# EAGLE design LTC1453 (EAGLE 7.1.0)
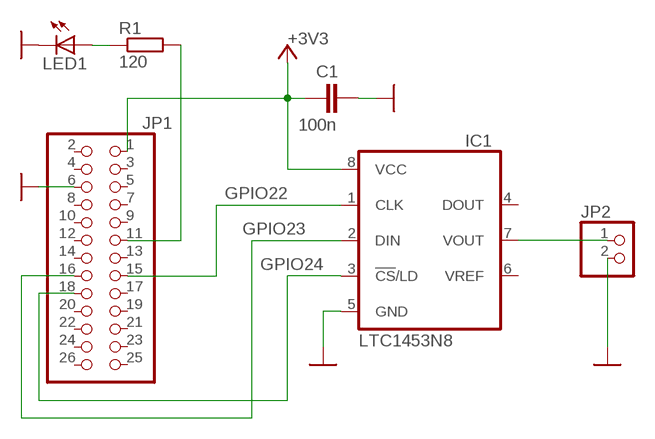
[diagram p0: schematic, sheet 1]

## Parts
C1  100n  C-EU025-024X044  [C025-024X044]
IC1  LTC1453N8  [DIL08]
JP1  PINHD-2X13  [2X13]
JP2  PINHD-1X2  [1X02]
LED1  LED5MM  [LED5MM]
R1  120  R-EU_0207/10  [0207/10]

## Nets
+3V3: C1.1 IC1.8(VCC) JP1.1
GND: C1.2 IC1.5(GND) JP1.6 JP2.2 LED1.K(C)
N$1: IC1.7(VOUT) JP2.1
N$3: IC1.3(!CS!/LD) JP1.18
N$4: IC1.1(CLK) JP1.15
N$5: IC1.2(DIN) JP1.16
N$6: LED1.A R1.1
N$7: JP1.11 R1.2
Unconnected: IC1.4(DOUT) IC1.6(VREF) JP1.2 JP1.3 JP1.4 JP1.5 JP1.7 JP1.8 JP1.9 JP1.10 JP1.12 JP1.13 JP1.14 JP1.17 JP1.19 JP1.20 JP1.21 JP1.22 JP1.23 JP1.24 JP1.25 JP1.26

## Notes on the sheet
- GPIO22
- GPIO23
- GPIO24

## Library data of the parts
C1 = rcl:C-EU: CAPACITOR, European symbol
IC1 = ltc145x:LTC145*: 12-Bit Rail-toRail A/D Micropower Converters; MPN: LTC1453CN8
JP1 = pinhead:PINHD-2X13: PIN HEADER
JP2 = pinhead:PINHD-1X2: PIN HEADER
LED1 = led:LED: LED
R1 = rcl:R-EU_: RESISTOR, European symbol

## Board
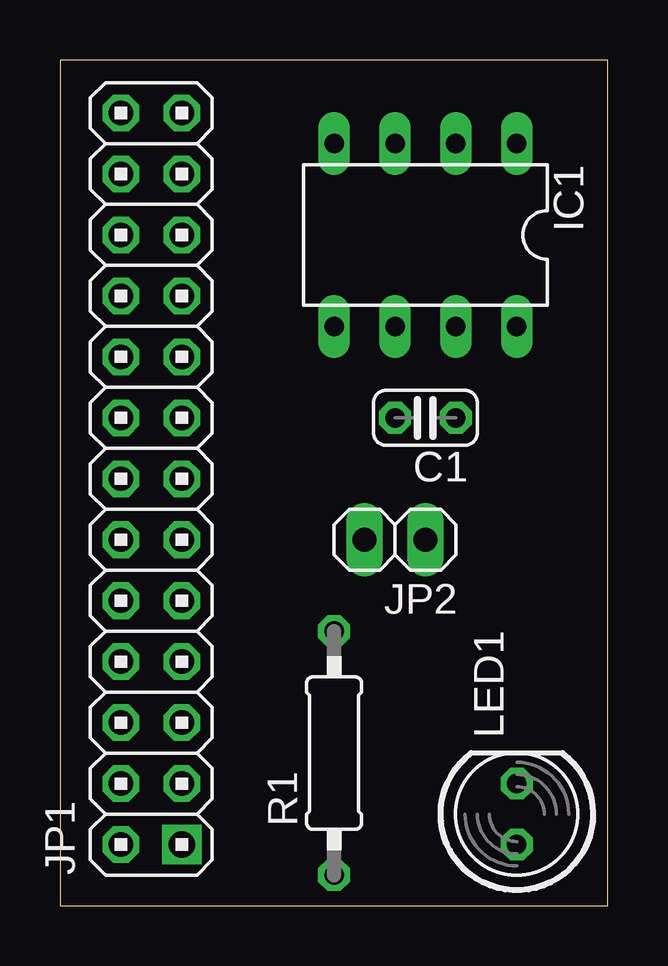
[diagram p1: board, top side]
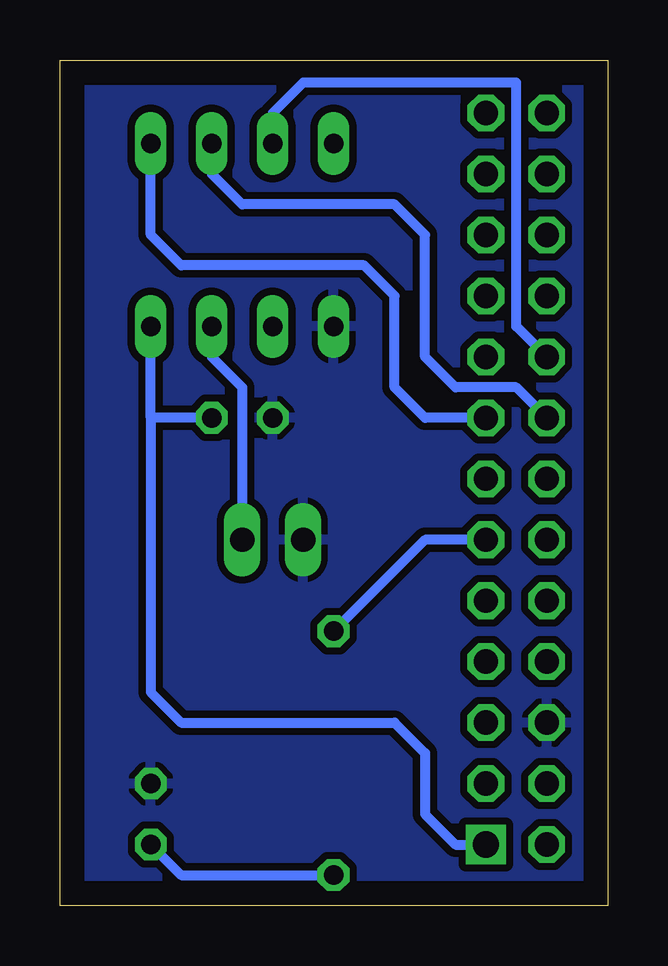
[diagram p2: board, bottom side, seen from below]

Size 22.84 x 35.23 mm. Coordinates in mm from the lower left corner, seen from the top.
Outline: 0,0 22.84,0 22.84,35.23 0,35.23 0,0
Copper layers (1*16): Top 0.035mm / dielectric 1.5mm / Bottom 0.035mm
Design rules "default": minimum track width 10mil, minimum drill 24mil, track to track 8mil, track to pad 8mil, pad to pad 8mil, via to via 8mil, smd to smd 8mil, copper to edge 40mil, drill to drill 8mil, minimum pad ring 10mil, minimum via ring 8mil, stop-mask expansion 4mil, vias tented up to drill 0mil, thermal gap 10mil

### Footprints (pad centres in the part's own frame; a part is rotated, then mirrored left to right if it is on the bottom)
C025-024X044 = drill 0.813 octagon: 1 -1.27,0; 2 1.27,0
DIL08 = drill 0.813 long: 1 -3.81,-3.81; 2 -1.27,-3.81; 3 1.27,-3.81; 4 3.81,-3.81; 5 3.81,3.81; 6 1.27,3.81; 7 -1.27,3.81; 8 -3.81,3.81
2X13 = drill 1.016 octagon: 1 -15.24,-1.27; 2 -15.24,1.27; 3 -12.7,-1.27; 4 -12.7,1.27; 5 -10.16,-1.27; 6 -10.16,1.27; 7 -7.62,-1.27; 8 -7.62,1.27; 9 -5.08,-1.27; 10 -5.08,1.27; 11 -2.54,-1.27; 12 -2.54,1.27; 13 0,-1.27; 14 0,1.27; 15 2.54,-1.27; 16 2.54,1.27; 17 5.08,-1.27; 18 5.08,1.27; 19 7.62,-1.27; 20 7.62,1.27; 21 10.16,-1.27; 22 10.16,1.27; 23 12.7,-1.27; 24 12.7,1.27; 25 15.24,-1.27; 26 15.24,1.27
1X02 = drill 1.016 long: 1 -1.27,0; 2 1.27,0
LED5MM = drill 0.813 octagon: A -1.27,0; K 1.27,0
0207/10 = drill 0.813 octagon: 1 -5.08,0; 2 5.08,0

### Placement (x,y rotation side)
C1  15.24,20.32 180 top
IC1  15.24,27.94 180 top
JP1  3.81,17.78 90 top
JP2  13.97,15.24 180 top
LED1  19.05,3.81 90 top
R1  11.43,6.35 90 top

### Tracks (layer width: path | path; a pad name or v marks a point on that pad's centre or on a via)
+3V3
  Bottom 0.406: 19.05,20.32 IC1.8 | 19.05,20.32 19.05,8.89 17.78,7.62 8.89,7.62 7.62,6.35 7.62,3.81 6.35,2.54 JP1.1 | C1.1 19.05,20.32
GND
  pour Bottom (isolate 0.305): 0,0 22.86,0 22.86,35.56 0,35.56
N$1
  Bottom 0.406: IC1.7 16.51,22.86 15.24,21.59 JP2.1
N$2  (via drill 1.1)
  other vias: 5.08,2.54
N$3
  Bottom 0.406: JP1.18 3.81,24.13 3.81,34.29 12.7,34.29 13.97,33.02 IC1.3
N$4
  Bottom 0.406: JP1.15 7.62,20.32 8.89,21.59 8.89,25.4 10.16,26.67 17.78,26.67 19.05,27.94 IC1.1
N$5
  Bottom 0.406: JP1.16 3.81,21.59 6.35,21.59 7.62,22.86 7.62,27.94 8.89,29.21 15.24,29.21 16.51,30.48 IC1.2
N$6
  Bottom 0.406: LED1.A 17.78,1.27 R1.1
N$7
  Bottom 0.406: JP1.11 7.62,15.24 R1.2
